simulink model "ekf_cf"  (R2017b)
settings: Solver=ode4  StartTime=0.0  StopTime=10.0  FixedStep=0.001  RelTol=1e-3  EnableMultiTasking=on
undefined symbols (not defined in the file or in its folder): RGBLED_COLOR_ENUM, RGBLED_MODE_ENUM
libraries: pixhawk_slib_sensors_actuators x4

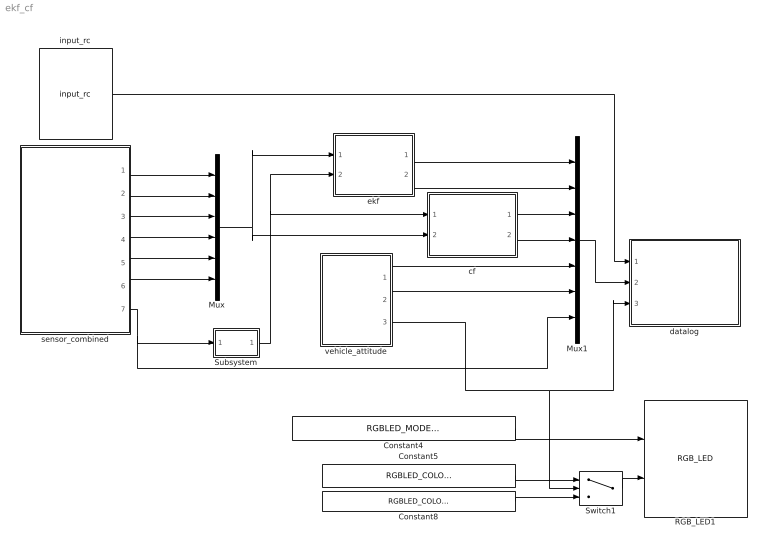
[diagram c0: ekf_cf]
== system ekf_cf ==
  Constant4 : Constant  Value=RGBLED_MODE_ENUM.SL_MODE_BLINK_NORMAL  OutDataTypeStr=Enum: RGBLED_MODE_ENUM
  Constant5 : Constant  Value=RGBLED_COLOR_ENUM.SL_COLOR_GREEN  OutDataTypeStr=Enum: RGBLED_COLOR_ENUM
  Constant8 : Constant  Value=RGBLED_COLOR_ENUM.SL_COLOR_RED  OutDataTypeStr=Enum: RGBLED_COLOR_ENUM
  Mux : Mux  Inputs=6
  Mux1 : Mux  Inputs=7
  RGB_LED1 : pixhawk_slib_sensors_actuators/RGB_LED  Description=|
      | This block gives the user control over various lighting modes of the RGB LED available on the PX4 hardware. 
      | This block accepts 2 inputs: Mode and Color.  These are enumeration data types.  You can find out what values are valid in the MATLAB command window by typing: 
      | Enumeration members for class 'RGBLED_COLOR_ENUM':
      |     SL_COLOR_OFF
      |     SL_COLOR_RED
      |     SL_COLOR_GREEN
      |     SL_COLOR_BLUE
      |     SL_C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
  Subsystem : Subsystem
  Switch1 : Switch  Criteria=u2 ~= 0  Threshold=1500
  cf : Subsystem
  datalog : Subsystem
  ekf : Subsystem
  input_rc : pixhawk_slib_sensors_actuators/input_rc  Description=|  sampletime=1/250  channel1=off  channel2=off  channel3=off  channel4=off  channel5=on  channel6=off  channel7=off  channel8=off  channel9=off  channel10=off  channel11=off  channel12=off  channel13=off  channel14=off  channel15=off  channel16=off  channel17=off  channel18=off  ch_count=off  rssi=off  rc_failsafe=off  rc_lost=off  rc_inputsource=off
      | RC Input Block
      | 
      | This block provides user input control to the model.
      | It uses the input_rc uORB topic.
      | 
      | The user has the ability to choose which channels are available as outputs from this block and also some optional outputs. These include 
      | Channels 1 through 18
      | double data type indicating the PWM value from the controller 
      | measured pulse widths for each of the supported channels 
      | Channel Count 
      | u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
  sensor_combined : Subsystem
  vehicle_attitude : Subsystem
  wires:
  sensor_combined/1(GyroX(p)) -> Mux/1
  sensor_combined/2(GyroY(q)) -> Mux/2
  sensor_combined/3(GyroZ(r)) -> Mux/3
  sensor_combined/4(AccelX) -> Mux/4
  sensor_combined/5(AccelY) -> Mux/5
  sensor_combined/6(AccelZ) -> Mux/6
  Mux/1 -> ekf/1(z), cf/2(z)
  sensor_combined/7(Ts) -> Mux1/7, Subsystem/1(Ts)
  Subsystem/1(dt) -> ekf/2(dt), cf/1(dt)
  vehicle_attitude/1(roll(phi)) -> Mux1/5
  vehicle_attitude/2(pitch(theta)) -> Mux1/6
  Mux1/1 -> datalog/2(data)
  input_rc/1 -> datalog/1(rc_input)
  Constant8/1 -> Switch1/3
  vehicle_attitude/3(en) -> datalog/3(datalog_flag), Switch1/2
  Constant4/1 -> RGB_LED1/1
  Constant5/1 -> Switch1/1
  Switch1/1 -> RGB_LED1/2
  cf/1(phi) -> Mux1/3
  cf/2(theta) -> Mux1/4
  ekf/1(phi) -> Mux1/1
  ekf/2(theta) -> Mux1/2

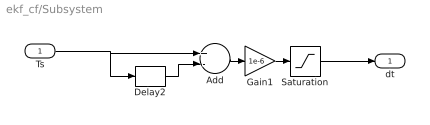
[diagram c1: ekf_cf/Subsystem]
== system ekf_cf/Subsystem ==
  Ts : Inport
  Add : Sum  Inputs=+-
  Delay2 : Delay  DelayLength=1
  Gain1 : Gain  Gain=1e-6
  Saturation : Saturate  UpperLimit=0.1  LowerLimit=0.001
  dt : Outport
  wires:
  Delay2/1 -> Add/2
  Saturation/1 -> dt/1
  Ts/1 -> Delay2/1, Add/1
  Gain1/1 -> Saturation/1
  Add/1 -> Gain1/1

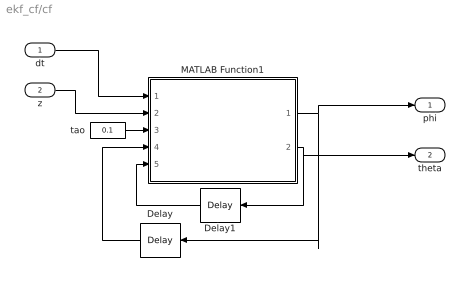
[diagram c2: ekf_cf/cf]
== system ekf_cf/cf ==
  dt : Inport
  z : Inport  Port=2
  Delay : Delay  DelayLength=1  InitialCondition=0
  Delay1 : Delay  DelayLength=1  InitialCondition=0
  MATLAB Function1 : MATLAB Function  TreatAsAtomicUnit=on
  tao : Constant  Value=0.1  OutDataTypeStr=single
  phi : Outport
  theta : Outport  Port=2
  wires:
  tao/1 -> MATLAB Function1/3(tao)
  MATLAB Function1/2(theta_cf) -> theta/1, Delay1/1
  MATLAB Function1/1(phi_cf) -> phi/1, Delay/1
  Delay1/1 -> MATLAB Function1/5(theta_cf_k)
  Delay/1 -> MATLAB Function1/4(phi_cf_k)
  z/1 -> MATLAB Function1/2(z)
  dt/1 -> MATLAB Function1/1(dt)

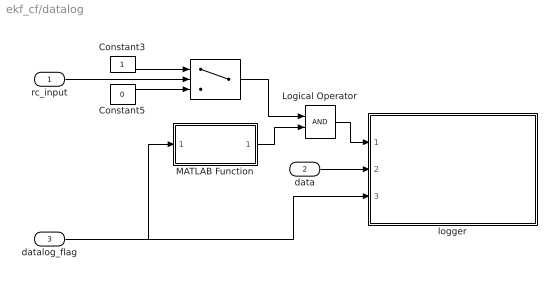
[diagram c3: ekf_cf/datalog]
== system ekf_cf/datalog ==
  rc_input : Inport
  data : Inport  Port=2
  datalog_flag : Inport  Port=3
  " " : Switch  Criteria=u2 > Threshold  Threshold=1600
  Constant3 : Constant
  Constant5 : Constant  Value=0
  Logical Operator : Logic  AllPortsSameDT=off  OutDataTypeStr=boolean
  MATLAB Function : MATLAB Function  TreatAsAtomicUnit=on
  logger : Subsystem  mask(Binary Logger){logfile=/fs/microsd/log/e4_ekf, cacheflag=off, numRecs=60000}
      mask prompts: cacheflag "Cache in Memory"; numRecs "Max Record Count"
      mask help: Log a vector of data to a file on the SD card If Cache in Memory is on data is written when en goes low or when max number of records specified is reached. Otherwise Max Number of Records is used to indicate when to performa an fflush out to file.
      mask init:
      | logname=uint8(logfile);
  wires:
  rc_input/1 -> " "/2
  data/1 -> logger/2(data)
  datalog_flag/1 -> logger/3(datalog_flag), MATLAB Function/1(datalog_flag)
  Constant3/1 -> " "/1
  Constant5/1 -> " "/3
  " "/1 -> Logical Operator/1
  MATLAB Function/1(en) -> Logical Operator/2
  Logical Operator/1 -> logger/1(en)

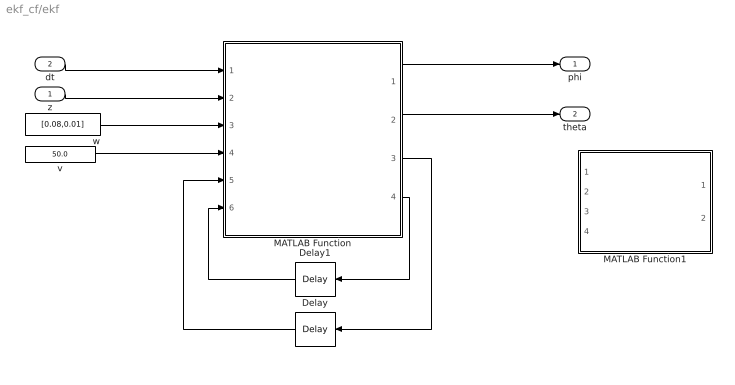
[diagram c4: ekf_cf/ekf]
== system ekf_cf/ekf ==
  z : Inport
  dt : Inport  Port=2
  Delay : Delay  DelayLength=1  InitialCondition=single([0, 0, 0, 0, 0, -1]')
  Delay1 : Delay  DelayLength=1  InitialCondition=single(eye(6, 6)*100)
  MATLAB Function : MATLAB Function  TreatAsAtomicUnit=on
  MATLAB Function1 : MATLAB Function  Commented=on  TreatAsAtomicUnit=on
  v : Constant  Value=50.0
  w : Constant  Value=[0.08,0.01]
  phi : Outport
  theta : Outport  Port=2
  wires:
  MATLAB Function/4(P_aposteriori) -> Delay1/1
  Delay/1 -> MATLAB Function/5(x_aposteriori_k)
  v/1 -> MATLAB Function/4(r)
  z/1 -> MATLAB Function/2(z)
  dt/1 -> MATLAB Function/1(dt)
  w/1 -> MATLAB Function/3(q)
  MATLAB Function/3(x_aposteriori) -> Delay/1
  Delay1/1 -> MATLAB Function/6(P_aposteriori_k)
  MATLAB Function/1(roll) -> phi/1
  MATLAB Function/2(pitch) -> theta/1

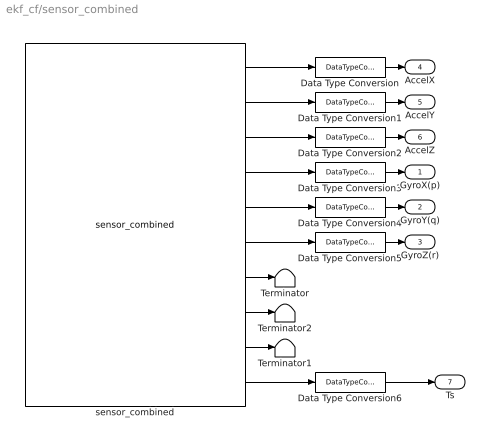
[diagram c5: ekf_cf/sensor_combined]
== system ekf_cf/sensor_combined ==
  Data Type Conversion{,1..6} (7 alike) : DataTypeConversion  OutDataTypeStr=single
  Terminator : Terminator
  Terminator1 : Terminator
  Terminator2 : Terminator
  sensor_combined : pixhawk_slib_sensors_actuators/sensor_combined  Description=|  sampletime=1/250  show_mag=off  show_acc=on  show_gyro=on  show_baro=off  show_ts=on
      | Sensor Combined Block
      | 
      | This block enables access to the various sensors available on the px4fmu-v2 hardware.  
      | The user can use these signals in the Simulink control model.  
      | The sample time needs to be provided in the mask dialog.  
      | Optional output ports can also be selected.  
      | Refer to the sample model: px4demo_attitude_control.slx
      | 
      | Signal definitions: 
      | Magnetometer (x,y,z) - single values – Mag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
  GyroX(p) : Outport
  GyroY(q) : Outport  Port=2
  GyroZ(r) : Outport  Port=3
  AccelX : Outport  Port=4
  AccelY : Outport  Port=5
  AccelZ : Outport  Port=6
  Ts : Outport  Port=7
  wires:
  sensor_combined/7 -> Terminator/1
  sensor_combined/1 -> Data Type Conversion/1
  sensor_combined/9 -> Terminator1/1
  sensor_combined/4 -> Data Type Conversion3/1
  Data Type Conversion/1 -> AccelX/1
  Data Type Conversion2/1 -> AccelZ/1
  Data Type Conversion5/1 -> GyroZ(r)/1
  Data Type Conversion3/1 -> GyroX(p)/1
  Data Type Conversion1/1 -> AccelY/1
  Data Type Conversion4/1 -> GyroY(q)/1
  sensor_combined/6 -> Data Type Conversion5/1
  sensor_combined/5 -> Data Type Conversion4/1
  sensor_combined/2 -> Data Type Conversion1/1
  sensor_combined/3 -> Data Type Conversion2/1
  Data Type Conversion6/1 -> Ts/1
  sensor_combined/8 -> Terminator2/1
  sensor_combined/10 -> Data Type Conversion6/1

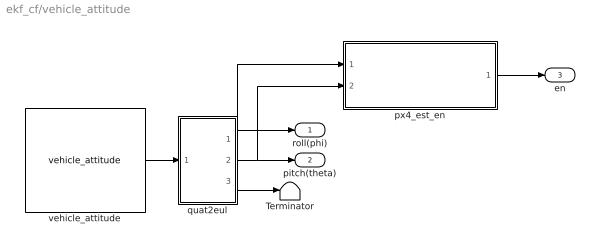
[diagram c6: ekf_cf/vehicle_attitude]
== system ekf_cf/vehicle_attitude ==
  Terminator : Terminator
  px4_est_en : MATLAB Function  TreatAsAtomicUnit=on
  quat2eul : MATLAB Function  TreatAsAtomicUnit=on
  vehicle_attitude : pixhawk_slib_sensors_actuators/vehicle_attitude  Description=|  sampletime=0.004  show_r=off  show_p=off  show_y=off  show_q=on  show_ts=off
      | This block gives access to the running service that calculates the vehicle’s attitude.  A uORB topic (vehicle_attitude (attitude measurements)) publisher MUST be running in order for this block to provide valid signal values.  The available ones as of v1.3 are: 
      | attitude_estimator_ekf – EKF-Extended Kalman Filter for attitude estimation 
      | attitude_estimator_so3 – SO(3)-attitude estimation by using 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
  roll(phi) : Outport
  pitch(theta) : Outport  Port=2
  en : Outport  Port=3
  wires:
  quat2eul/1(phi) -> px4_est_en/1(roll), roll(phi)/1
  quat2eul/2(theta) -> px4_est_en/2(pitch), pitch(theta)/1
  quat2eul/3(psi) -> Terminator/1
  vehicle_attitude/1 -> quat2eul/1(q)
  px4_est_en/1(px4_att_est_ok) -> en/1

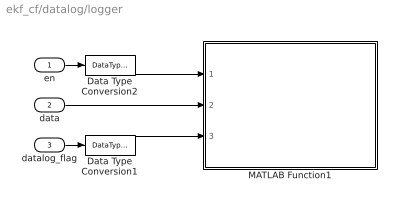
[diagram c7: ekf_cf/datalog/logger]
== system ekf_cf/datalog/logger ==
  en : Inport
  data : Inport  Port=2
  datalog_flag : Inport  Port=3
  Data Type Conversion1 : DataTypeConversion  OutDataTypeStr=boolean
  Data Type Conversion2 : DataTypeConversion  OutDataTypeStr=boolean
  MATLAB Function1 : MATLAB Function  TreatAsAtomicUnit=on
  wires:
  data/1 -> MATLAB Function1/2(data)
  Data Type Conversion2/1 -> MATLAB Function1/1(en)
  en/1 -> Data Type Conversion2/1
  datalog_flag/1 -> Data Type Conversion1/1
  Data Type Conversion1/1 -> MATLAB Function1/3(datalog_flag)

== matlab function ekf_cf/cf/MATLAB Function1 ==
function [ phi_cf, theta_cf ] = Attitude_cf(dt, z, tao, phi_cf_k, theta_cf_k)
%Function description:
%  complementary filter  for attitude estimation.
%Input:
%  dt: sampling time, unit: s
%  z: three-axis gyroscope and three-axis accelerometer data, [gx, gy, gz, ax, ay, az]', unit: rad/s, m/s2
%  phi_cf_k, theta_cf_k: angle value of the previous sampling, unit: rad
%  tao: filter coefficient
%Output:
%  phi_cf, theta_cf: attitude angle, unit: rad

    gx = z(1); gy = z(2);
    ax = z(4); ay = z(5); az = z(6);
    
    % calculate Euler angles using accelerometer data
    g = sqrt(ax*ax + ay*ay + az*az);
    theta_am = asin(ax/g);
    phi_am = -asin(ay/(g*cos(theta_am)));
    
    % complementary filtering
    theta_cf = tao/(tao + dt)*(theta_cf_k + gy*dt) + dt/(tao + dt)*theta_am;
    phi_cf = tao/(tao + dt)*(phi_cf_k + gx*dt) + dt/(tao + dt)*phi_am;
end

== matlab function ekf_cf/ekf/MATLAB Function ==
function [roll, pitch, x_aposteriori, P_aposteriori] = Attitude_ekf( dt, z, q, r, x_aposteriori_k, P_aposteriori_k)
%Function description:
%  Extended Kalman Filtering Method for State Estimation
%Input:
%  dt: Update Cycle
%  z: Measured value (6,1)
%  q: System noise,r:Measuring noise
%  x_aposteriori_k: State estimate at the last moment (6,1)
%  P_aposteriori_k: Estimate covariance at the last moment (6,6)
%Output:
%  x_aposteriori：State estimate of current time (6,1)
%  P_aposteriori：Estimated covariance at the current moment (6,6)
%  roll、pitch：Euler angle, unit: rad


w_m = z(1 : 3);  %Angular velocity measurement
a_m = z(4 : 6);  %Acceleration measurement
g = norm(a_m, 2);  %Gravity acceleration
%   w_x_=[ 0,-(wz-bzg, wy-byg;
%         wz-bzg, 0 ,-(wx-bxg);
%         -(wy-byg), wx-bxg, 0];
    w_x_ = [0, -(w_m(3) - x_aposteriori_k(3)), w_m(2) - x_aposteriori_k(2);
         w_m(3) - x_aposteriori_k(3), 0, -(w_m(1) - x_aposteriori_k(1));
         -(w_m(2) - x_aposteriori_k(2)), w_m(1) - x_aposteriori_k(1), 0];
     
	bCn = eye(3, 3) - w_x_*dt;
% update a priori state matrix
  x_apriori = zeros(1, 6);
  x_apriori(1: 3) = x_aposteriori_k(1 : 3);  %Angular velocity drift
  x_apriori(4 : 6) = bCn*x_aposteriori_k(4 : 6);  %Acceleration normalized value
  %[x]x
  x_aposteriori_k_x = [0, -x_aposteriori_k(6), x_aposteriori_k(5);
                        x_aposteriori_k(6), 0, -x_aposteriori_k(4);
                        -x_aposteriori_k(5), x_aposteriori_k(4), 0];
% update state transition matrix
 PHI = [eye(3, 3), zeros(3, 3);
         -x_aposteriori_k_x*dt,bCn];
 GAMMA = [eye(3, 3)*dt, zeros(3, 3);
             zeros(3, 3), -x_aposteriori_k_x*dt];
  % prediction error covariance matrix
  Q = [eye(3, 3)*q(1), zeros(3, 3);
     zeros(3, 3), eye(3, 3)*q(2)];
 P_apriori = PHI*P_aposteriori_k*PHI' + GAMMA*Q*GAMMA';
%%
%Kalman gain
 R = eye(3, 3)*r(1);
 H_k = [zeros(3, 3), g*eye(3, 3)];
 K_k = (P_apriori*H_k')/(H_k*P_apriori*H_k' + R);
  % state estimation matrix
  x_aposteriori = x_apriori' + K_k*(a_m - H_k*x_apriori');
  % estimated error covariance
  P_aposteriori = (eye(6, 6) - K_k*H_k)*P_apriori;
 %%
  % calculate roll, pitch
  k = -x_aposteriori(4 : 6) /norm(x_aposteriori(4 : 6), 2);
  
  roll = atan2(k(2) , k(3));
  pitch = -asin(k(1));
end

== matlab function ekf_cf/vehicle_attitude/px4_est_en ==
function px4_att_est_ok = px4_est_en(roll, pitch)

if abs(roll) < 0.000001 && abs(pitch) < 0.000001
    px4_att_est_ok = false;
else
    px4_att_est_ok = true;
end

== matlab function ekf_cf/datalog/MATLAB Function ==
function en = fcn(datalog_flag)

persistent count;
if isempty(count)
    count=0;
end

if datalog_flag
    count=count+1;
end
if count>60000
    en = false;
    count=0;
else
    en = true;
end

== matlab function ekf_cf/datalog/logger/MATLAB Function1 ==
%% Binary Logger
% Note: All data needs to be of the same type (e.g. double)
% Header information format:
%           String "MWLOGV##"
%           Time/Date 4 bytes (time())
%           Number of Signals per record Logged 1 byte (256 max)
%           Data Type of Signals Logged  1 byte (1-10)
%           Number of bytes per record 2 bytes (65535 max)
% This does NOT include the number of data sets logged.  
% i.e. The Reader is responsible for reading until EOF.
% MathWorks Pilot Engineering 2015
% Steve Kuznicki
function binary_logger(en, data, datalog_flag, logname, cacheflag, numRecs)
%#codegen
    persistent fp isflushed isopen count lognumstr elem_size vect_size
    coder.cinclude('<stdio.h>');
    coder.cinclude('<time.h>');
    
    if isempty(count)
        count = uint32(0);
        lognumstr = 65;
        isopen = false;
        fp = coder.opaque('FILE*', 'NULL');
        isflushed = false;
        elem_size = uint16(1);
        vect_size = coder.const(uint8(numel(data)));
        if cacheflag == true
            %datastored = zeros(numRecs*uint32(coder.const(numel(data))), 1, 'like', data);
        end
    end

    if (en)
        if isopen == false
            [elsize, eltype] = get_elem_size(data);
            elem_size = coder.const(uint16(elsize));
            elem_type = coder.const(uint8(eltype));
            vect_size = coder.const(uint8(numel(data)));
            coder.ceval('printf',['OPENING file %s vect_size %d elem_size %d numRecs %d %c' uint8(0)], ...
                [logname, '_', char(lognumstr), '.bin', int8(0)], uint32(vect_size), uint32(elem_size), uint32(numRecs), uint8(10));
            fp = coder.ceval('fopen', [logname, '_', char(lognumstr), '.bin', int8(0)], ['wb', int8(0)]);
            lognumstr = lognumstr + 1;
            isflushed = false;
            count = uint32(0);
            isopen = true;
            % Write header information here
            % header token + version
            mlStrVer = 'MWLOGV01';
            coder.ceval('fwrite', coder.rref(mlStrVer), uint32(1), length(mlStrVer), fp);
            % date/time
            tm = uint32(0);
            tmptr = uint32(0);
            tm = coder.ceval('time',coder.wref(tmptr));
            coder.ceval('fwrite', coder.rref(tm), uint32(4), uint32(1), fp);
            % number of elements in each record
            coder.ceval('fwrite', coder.rref(vect_size), uint32(1), uint32(1), fp);
            % data type of the elements
            coder.ceval('fwrite', coder.rref(elem_type), uint32(1), uint32(1), fp);
            % size of each record in bytes
            recSize = elem_size * uint16(vect_size);
            coder.ceval('fwrite', coder.rref(recSize), uint32(2), uint32(1), fp);
        end
        % cache data in memory or use fwrite
        if cacheflag == true
            addr = (count*uint32(vect_size))+1;
            for idx = 1:vect_size
                %datastored(addr) = data(idx);
                addr = addr + 1;
            end
            count = count + uint32(1);
        else
            if  datalog_flag
                coder.ceval('fwrite', coder.rref(data), elem_size, vect_size, fp);
                count = count + uint32(1);
            end
        end
        
        % check for data count limit
        if count >= numRecs
            if cacheflag
                for idx = 1:count*uint32(vect_size)
                    %coder.ceval('fwrite', coder.rref(datastored(idx)), elem_size, uint32(1), fp);
                end
            end
            coder.ceval('fflush', fp);
            isflushed = false;
            count = uint32(0);
        end
    else
        if isopen == true
            if ~isflushed 
                coder.ceval('printf',['CLOSING file. count = %d %c' uint8(0)], uint32(count), uint8(10));
                if cacheflag
                    count = count + uint32(1);
                    for idx = 1:count*uint32(vect_size)
                        %coder.ceval('fwrite', coder.rref(datastored(idx)), elem_size, uint32(1), fp);
                    end
                end
                coder.ceval('fflush', fp);
                isflushed = true;
            end
            coder.ceval('fclose', fp);
        end
        isopen = false;
        count = uint32(0);
    end
end

% return the size of the element in bytes
function [elem_size, dtype] = get_elem_size(data)
    switch(class(data))
        case 'double'
            elem_size = 8;
            dtype = 1;
        case 'single'
            elem_size = 4;
            dtype = 2;
        case 'int32'
            elem_size = 4;
            dtype = 3;
        case 'uint32'
            elem_size = 4;
            dtype = 4;
        case 'int16'
            elem_size = 2;
            dtype = 5;
        case 'uint16'
            elem_size = 2;
            dtype = 6;
        case 'int8'
            elem_size = 1;
            dtype = 7;
        case 'uint8'
            elem_size = 1;
            dtype = 8;
        case 'logical'
            elem_size = 1;
            dtype = 9;
        case 'embedded.fi'
            nt = numerictype(data);
            elem_size = 2^ceil(log2(ceil(nt.WordLength / 8)));
            dtype = 10;
    end
    if ~isreal(data)
        elem_size = elem_size*2;
    end
    
    elem_size = uint16(elem_size);
    dtype = uint8(dtype);
end

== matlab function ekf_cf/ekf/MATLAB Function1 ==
function [roll, pitch] = Attitude_ekf( dt, z, q, r)
%Function description:
%  Extended Kalman Filtering Method for State Estimation
%Input:
%  dt: Update Cycle
%  z: Measured value (6,1)
%  q: System noise,r:Measuring noise
%  x_aposteriori_k: State estimate at the last moment (6,1)
%  P_aposteriori_k: Estimate covariance at the last moment (6,6)
%Output:
%  x_aposteriori：State estimate of current time (6,1)
%  P_aposteriori：Estimated covariance at the current moment (6,6)
%  roll、pitch：Euler angle, unit: rad

persistent x_aposteriori;
if  isempty(x_aposteriori)
  x_aposteriori = single([0, 0, 0, 0, 0, -1]');
end
persistent P_aposteriori;
if  isempty(P_aposteriori)
  P_aposteriori = single(eye(6, 6)*100);
end

x_aposteriori_k = x_aposteriori;
P_aposteriori_k = P_aposteriori;

w_m = z(1 : 3);  %Angular velocity measurement
a_m = z(4 : 6);  %Acceleration measurement
g = norm(a_m, 2);  %Gravity acceleration
%   w_x_=[ 0,-(wz-bzg, wy-byg;
%         wz-bzg, 0 ,-(wx-bxg);
%         -(wy-byg), wx-bxg, 0];
    w_x_ = [0, -(w_m(3) - x_aposteriori_k(3)), w_m(2) - x_aposteriori_k(2);
         w_m(3) - x_aposteriori_k(3), 0, -(w_m(1) - x_aposteriori_k(1));
         -(w_m(2) - x_aposteriori_k(2)), w_m(1) - x_aposteriori_k(1), 0];
     
	bCn = eye(3, 3) - w_x_*dt;
% update a priori state matrix
  x_apriori = zeros(1, 6);
  x_apriori(1: 3) = x_aposteriori_k(1 : 3);  %Angular velocity drift
  x_apriori(4 : 6) = bCn*x_aposteriori_k(4 : 6);  %Acceleration normalized value
  %[x]x
  x_aposteriori_k_x = [0, -x_aposteriori_k(6), x_aposteriori_k(5);
                        x_aposteriori_k(6), 0, -x_aposteriori_k(4);
                        -x_aposteriori_k(5), x_aposteriori_k(4), 0];
% update state transition matrix
 PHI = [eye(3, 3), zeros(3, 3);
         -x_aposteriori_k_x*dt,bCn];
 GAMMA = [eye(3, 3)*dt, zeros(3, 3);
             zeros(3, 3), -x_aposteriori_k_x*dt];
  % prediction error covariance matrix
  Q = [eye(3, 3)*q(1), zeros(3, 3);
     zeros(3, 3), eye(3, 3)*q(2)];
 P_apriori = PHI*P_aposteriori_k*PHI' + GAMMA*Q*GAMMA';
%%
%Kalman gain
 R = eye(3, 3)*r(1);
 H_k = [zeros(3, 3), g*eye(3, 3)];
 K_k = (P_apriori*H_k')/(H_k*P_apriori*H_k' + R);
  % state estimation matrix
  x_aposteriori = x_apriori' + K_k*(a_m - H_k*x_apriori');
  % estimated error covariance
  P_aposteriori = (eye(6, 6) - K_k*H_k)*P_apriori;
 %%
  % calculate roll, pitch
  k = -x_aposteriori(4 : 6) /norm(x_aposteriori(4 : 6), 2);
  
  roll = atan2(k(2) , k(3));
  pitch = -asin(k(1));
end

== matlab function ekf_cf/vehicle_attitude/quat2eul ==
function [phi,theta,psi] = quat2eul(q)
% Conversion from Quaternion to Euler angles based on the PX4 Firmware
% v1.6.5 release.
% 
% Quaternion -> DCM -> Euler Angles
% INPUT:
%   q: Quaternion vector of the format: (a + bi + cj + dk)
% OUTPUT:
%   [phi,theta,psi]: Euler angles in radians.
% 
 
    a = q(1);
    b = q(2);
    c = q(3);
    d = q(4);

    aSq = a*a;
    bSq = b*b;
    cSq = c*c;
    dSq = d*d;

    d_pi2 = pi/2;

    % quaternion_to_dcm
    dcm00 = aSq + bSq - cSq - dSq;
    % dcm01 = 2*(b*c - a*d);
    dcm02 = 2*(a*c + b*d);
    dcm10 = 2*(b*c + a*d);
    % dcm11 = aSq - bSq + cSq - dSq;
    dcm12 = 2*(c*d - a*b);
    dcm20 = 2*(b*d - a*c);
    dcm21 = 2*(a*b + c*d);
    dcm22 = aSq - bSq - cSq + dSq;

    % dcm_to_euler
    theta = asin(-dcm20);
    if abs(theta - d_pi2) < 1.0e-3
        phi = single(0.0);
        psi = atan2(dcm12, dcm02);
    elseif abs(theta + d_pi2) < 1.0e-3
        phi = single(0.0);
        psi = atan2(-dcm12, -dcm02);
    else
        phi = atan2(dcm21, dcm22);
        psi = atan2(dcm10, dcm00);
    end

end
